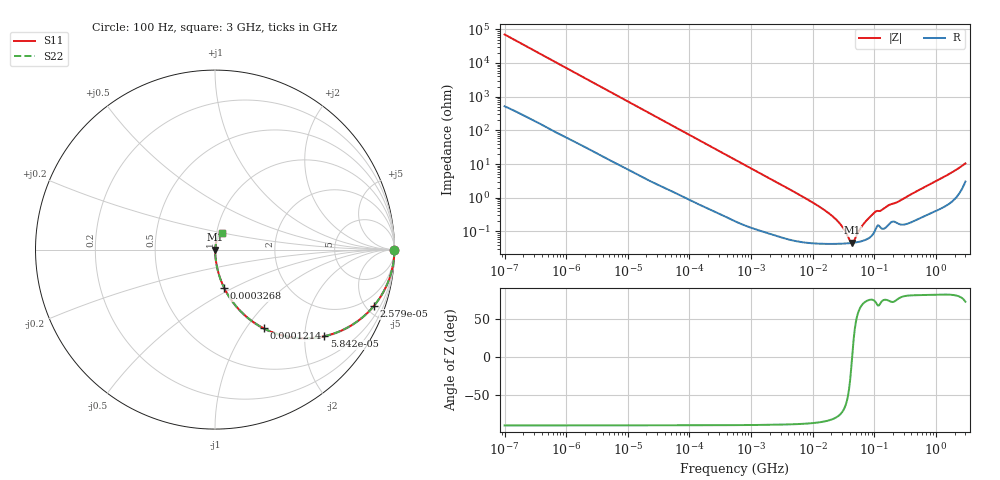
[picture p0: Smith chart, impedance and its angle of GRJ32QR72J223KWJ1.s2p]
!Murata Part Number: GRJ32QR72J223KWJ1
!These Parameters are Measured in Series Mode Connection
!Data Generated on Jun 19, 2026
!  o--ll--o
!Port1  Port2
!  o------o
!Operation Temp=25[degC], DC Bias Voltage=0[V]
!Freq. Start=100[Hz] Stop=3[GHz] 401[Steps]
# Hz S RI R 50
!Freq.(Hz) S11(Real) S11(Imag) S21(Real) S21(Imag) S12(Real) S12(Imag) S22(Real) S22(Imag)
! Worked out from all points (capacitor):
!   401 points, 100 Hz to 3 GHz, reference 50 ohm
!   read as one part in series: C = 22.5 nF near 109 Hz
!   lowest |Z| = 46.2 mohm at 44.18 MHz (marker M1)
!   series resonance near 43.52 MHz, so ESL is about 590 pH
!   S11 on the Smith chart (normalised r, x): 100 Hz: open; 25.79 kHz: 1.06, -5.64; 58.42 kHz: 1.03, -2.50; 121.4 kHz: 1.01, -1.21; 326.8 kHz: 1.01, -0.45; 3 GHz: 1.06, +0.20
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100  1 -0.00142  1.25e-05 0.00142  1.25e-05 0.00142  1 -0.00142
1788  0.9992 -0.0249  0.000846 0.0249  0.000846 0.0249  0.9992 -0.0249
8066  0.9867 -0.11  0.0133 0.11  0.0133 0.11  0.9867 -0.11
25785  0.886 -0.3129  0.114 0.3129  0.114 0.3129  0.886 -0.3129
31977  0.8359 -0.3652  0.1641 0.3652  0.1641 0.3652  0.8359 -0.3652
58416  0.6094 -0.4823  0.3906 0.4823  0.3906 0.4823  0.6094 -0.4823
121426  0.2707 -0.4384  0.7293 0.4384  0.7293 0.4384  0.2707 -0.4384
194955  0.1285 -0.3282  0.8715 0.3282  0.8715 0.3282  0.1285 -0.3282
326774  0.0516 -0.2144  0.9484 0.2144  0.9484 0.2144  0.0516 -0.2144
547723  0.02 -0.1329  0.98 0.1329  0.98 0.1329  0.02 -0.1329
1677156  0.00293 -0.0445  0.9971 0.0445  0.9971 0.0445  0.00293 -0.0445
9794414  0.000499 -0.00736  0.9995 0.00736  0.9995 0.00736  0.000499 -0.00736
2.316512e7  0.000432 -0.00235  0.9996 0.00235  0.9996 0.00235  0.000432 -0.00235
2.999103e7  0.000435 -0.00133  0.9996 0.00133  0.9996 0.00133  0.000435 -0.00133
4.0536e7  0.00045 -0.000249  0.9995 0.000249  0.9995 0.000249  0.00045 -0.000249
4.418008e7  0.000458 5.37e-05  0.9995 -5.37e-05  0.9995 -5.37e-05  0.000458 5.37e-05
6.508213e7  0.000529 0.00147  0.9995 -0.00147  0.9995 -0.00147  0.000529 0.00147
8.79653e7  0.000711 0.0028  0.9993 -0.0028  0.9993 -0.0028  0.000711 0.0028
1.044919e8  0.00115 0.00368  0.9988 -0.00368  0.9988 -0.00368  0.00115 0.00368
1.751444e8  0.00171 0.0059  0.9983 -0.0059  0.9983 -0.0059  0.00171 0.0059
2.471375e8  0.00174 0.00754  0.9983 -0.00754  0.9983 -0.00754  0.00174 0.00754
3e9  0.0384 0.0935  0.9616 -0.0935  0.9616 -0.0935  0.0384 0.0935
